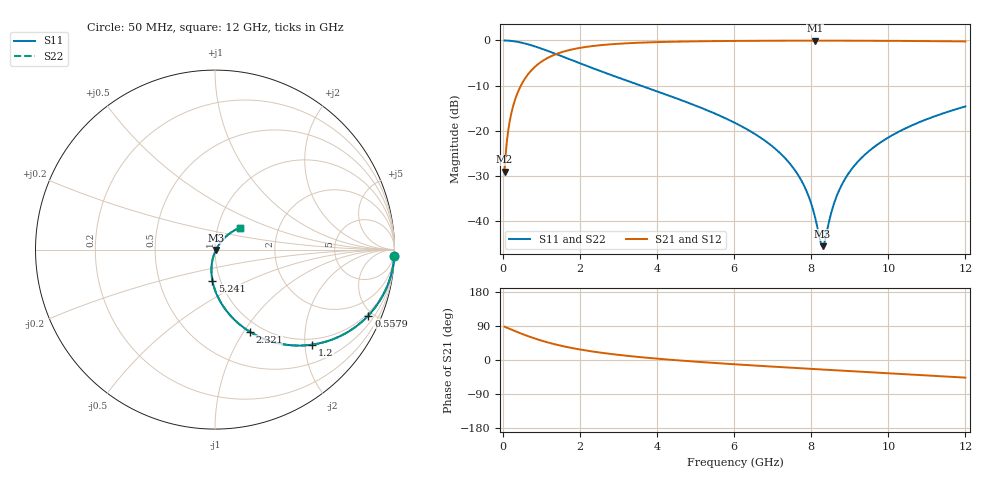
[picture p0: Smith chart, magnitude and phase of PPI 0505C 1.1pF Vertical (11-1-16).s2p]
# GHz S MA R 50
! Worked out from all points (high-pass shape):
!   1601 points, 50 MHz to 12 GHz, reference 50 ohm
!   highest |S21| = -0.05 dB at 8.101 GHz (marker M1); lowest = -29.1 dB at 50 MHz (marker M2)
!   |S21| within 3 dB of the highest: 1.378 GHz to end of sweep
!   lowest |S11| = -45.5 dB at 8.296 GHz (marker M3), VSWR 1.01, Z = 50.5 - j0.232 ohm
!   |S11| at or under -10 dB: 3.585 GHz to end of sweep
!   |S22| runs from -45.5 to 0.0 dB; largest |S21 - S12| = 0
!   S11 on the Smith chart (normalised r, x): 50 MHz: 1, -53; 557.9 MHz: 0.87, -4.71; 1.2 GHz: 0.87, -2.16; 2.321 GHz: 0.88, -1.06; 5.241 GHz: 0.92, -0.33; 12 GHz: 1.28, +0.33
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0.05  0.9994 -2.2  0.03523 87.8  0.03523 87.8  0.9994 -2.2
0.1545625  0.9941 -6.7  0.1084 83.3  0.1084 83.3  0.9941 -6.7
0.2367188  0.9863 -10.2  0.1647 79.8  0.1647 79.8  0.9863 -10.2
0.3711563  0.9672 -15.8  0.2535 74.1  0.2535 74.1  0.9672 -15.8
0.557875  0.9299 -23.3  0.3671 66.7  0.3671 66.7  0.9299 -23.3
1.200187  0.7572 -44.4  0.6516 45.5  0.6516 45.5  0.7572 -44.4
2.044156  0.5498 -62.7  0.8328 27.0  0.8328 27.0  0.5498 -62.7
2.3205  0.4958 -67.1  0.8657 22.6  0.8657 22.6  0.4958 -67.1
4.038312  0.27 -86.0  0.9591 3.3  0.9591 3.3  0.27 -86.0
5.240781  0.1732 -94.8  0.9805 -6.1  0.9805 -6.1  0.1732 -94.8
6.025  0.1224 -99.4  0.9878 -11.4  0.9878 -11.4  0.1224 -99.4
7.3395  0.04907 -103.8  0.9935 -19.5  0.9935 -19.5  0.04907 -103.8
7.742813  0.0284 -101.7  0.9941 -21.9  0.9941 -21.9  0.0284 -101.7
8.019156  0.01485 -93.1  0.9942 -23.5  0.9942 -23.5  0.01485 -93.1
8.101313  0.01108 -86.0  0.9942 -24.0  0.9942 -24.0  0.01108 -86.0
8.23575  0.006086 -54.7  0.9942 -24.8  0.9942 -24.8  0.006086 -54.7
8.2955  0.0053 -25.7  0.9942 -25.1  0.9942 -25.1  0.0053 -25.7
8.624125  0.01717 44.5  0.9939 -27.0  0.9939 -27.0  0.01717 44.5
8.907937  0.03081 50.9  0.9934 -28.7  0.9934 -28.7  0.03081 50.9
9.371  0.05341 52.4  0.9922 -31.3  0.9922 -31.3  0.05341 52.4
10.01331  0.08501 50.9  0.9897 -35.0  0.9897 -35.0  0.08501 50.9
12  0.1862 41.3  0.9747 -46.5  0.9747 -46.5  0.1862 41.3
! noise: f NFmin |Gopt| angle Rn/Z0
0.05  0.0011  0.967  1.558  0.007547
1.372  0.005838  0.7691  6.282  0.005135
2.701  0.009202  0.7173  9.867  0.00639
4.031  0.01218  0.687  13.54  0.007459
5.36  0.015  0.6669  17.22  0.008456
6.682  0.01773  0.6535  20.83  0.009436
8.012  0.02049  0.6447  24.4  0.01046
9.341  0.02331  0.6399  27.9  0.01155
10.67  0.02625  0.6385  31.33  0.01275
12  0.02936  0.64  34.68  0.0141
